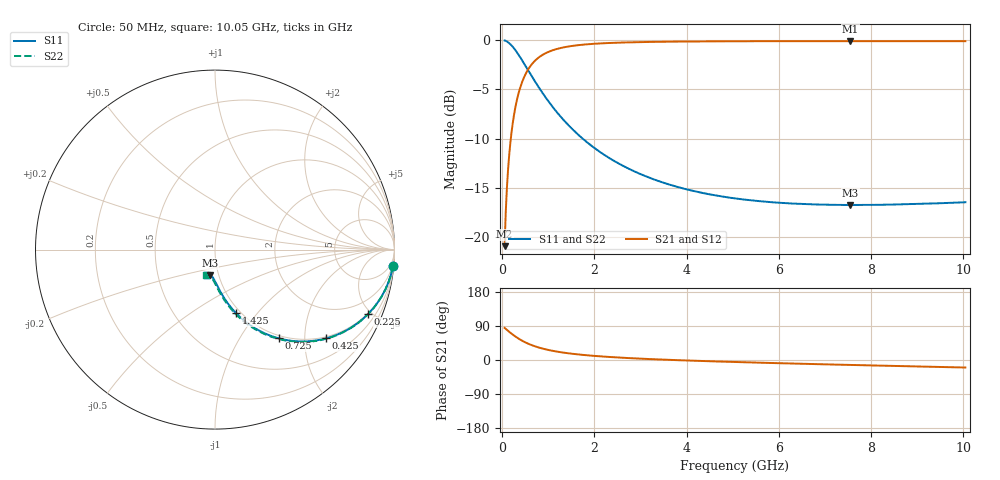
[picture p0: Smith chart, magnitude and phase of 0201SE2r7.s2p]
! AVX Thin Film Operation		Date: August 2001
! Description: Accu-P® Series, Thin Film, SMD, RF Capacitor
! Part Number: 02013J2R7ABW
! 50 MHz  -  10.05 GHz
! Serial Measurements
# mhz S db R 50
!	S11		S21		S12		S22
!	dB	Phase	dB	Phase	dB	Phase	dB	Phase
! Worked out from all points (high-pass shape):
!   401 points, 50 MHz to 10.05 GHz, reference 50 ohm
!   highest |S21| = -0.10 dB at 7.55 GHz (marker M1); lowest = -20.9 dB at 50 MHz (marker M2)
!   |S21| within 3 dB of the highest: 544 MHz to end of sweep
!   lowest |S11| = -16.7 dB at 7.55 GHz (marker M3), VSWR 1.34, Z = 45.3 - j13.3 ohm
!   |S11| at or under -10 dB: 1.747 GHz to end of sweep
!   |S22| runs from -16.7 to 0.0 dB; largest |S21 - S12| = 0
!   S11 on the Smith chart (normalised r, x): 50 MHz: 1, -22; 225 MHz: 0.96, -4.79; 425 MHz: 0.95, -2.54; 725 MHz: 0.95, -1.50; 1.425 GHz: 0.95, -0.78; 10.05 GHz: 0.87, -0.26
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50  -0.04 -5.3  -20.89 84.7  -20.89 84.7  -0.04 -5.3
75  -0.08 -7.9  -17.42 82.0  -17.42 82.0  -0.08 -8.0
125  -0.22 -13.1  -13.12 76.9  -13.12 76.9  -0.22 -13.2
150  -0.31 -15.6  -11.63 74.4  -11.63 74.4  -0.31 -15.7
175  -0.42 -18.0  -10.40 71.9  -10.40 71.9  -0.42 -18.1
225  -0.67 -22.7  -8.47 67.2  -8.47 67.2  -0.67 -22.9
325  -1.29 -31.3  -5.91 58.6  -5.91 58.6  -1.29 -31.5
425  -2.01 -38.6  -4.31 51.3  -4.31 51.3  -2.01 -38.8
575  -3.17 -47.4  -2.87 42.3  -2.87 42.3  -3.17 -47.8
725  -4.30 -54.3  -2.02 35.5  -2.02 35.5  -4.30 -54.7
875  -5.37 -59.6  -1.49 30.1  -1.49 30.1  -5.37 -60.1
1025  -6.36 -63.8  -1.15 25.8  -1.15 25.8  -6.36 -64.4
1425  -8.57 -71.7  -0.66 17.8  -0.66 17.8  -8.57 -72.5
1725  -9.91 -75.7  -0.47 13.7  -0.47 13.7  -9.91 -76.7
2500  -12.45 -82.5  -0.26 6.7  -0.26 6.7  -12.45 -83.9
3400  -14.31 -87.5  -0.17 1.4  -0.17 1.4  -14.31 -89.3
4150  -15.30 -90.7  -0.14 -1.9  -0.14 -1.9  -15.30 -92.7
5050  -16.05 -93.9  -0.12 -5.3  -0.12 -5.3  -16.05 -96.1
6725  -16.65 -99.1  -0.10 -10.7  -0.10 -10.7  -16.66 -101.4
7550  -16.72 -101.5  -0.10 -13.1  -0.10 -13.1  -16.72 -103.7
8400  -16.68 -103.8  -0.10 -15.4  -0.10 -15.4  -16.68 -106.1
10050  -16.44 -108.2  -0.11 -19.9  -0.11 -19.9  -16.44 -110.4
